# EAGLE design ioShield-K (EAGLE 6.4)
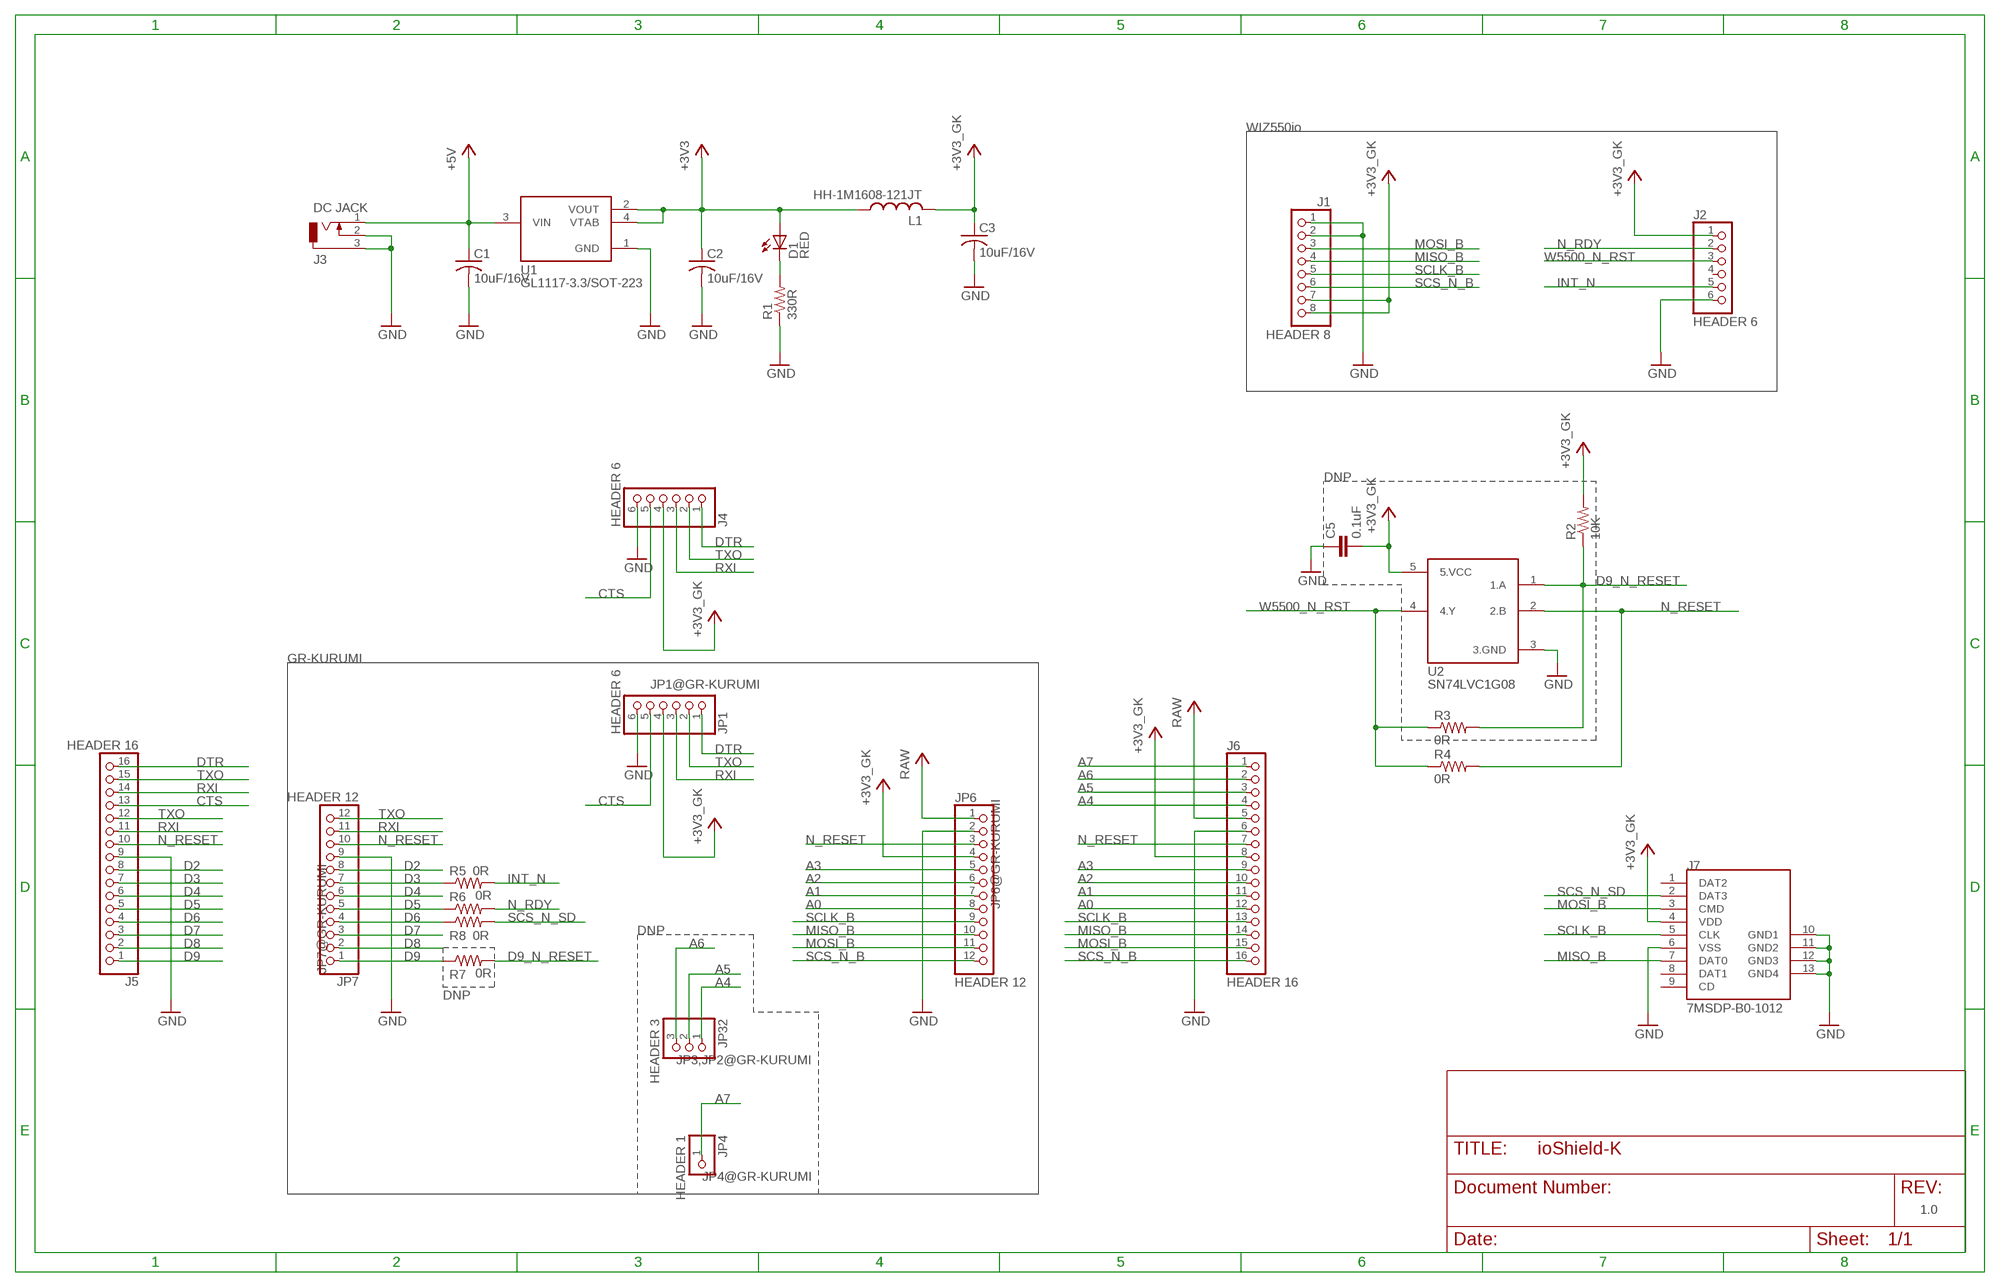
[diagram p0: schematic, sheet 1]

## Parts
C1  10uF/16V  CT-A(3216)  [CT-A(3216)]
C2  10uF/16V  CT-A(3216)  [CT-A(3216)]
C3  10uF/16V  CT-A(3216)  [CT-A(3216)]
C5  0.1uF  C1608  [C1608]
D1  RED  LED1608  [CHIP-LED1608]
J1  HEADER 8  HEADER8  [HEADER1X8]
J2  HEADER 6  HEADER6  [HEADER1X6]
J3  DC JACK  DC-005  [DC-005-PACK]
J4  HEADER 6  HEADER6  [HEADER1X6]
J5  HEADER 16  HEADER16  [HEADER1X16]
J6  HEADER 16  HEADER16  [HEADER1X16]
J7  7MSDP-B0-1012  [MICROSD_HC]
JP1  HEADER 6  HEADER6  [HEADER1X6]
JP4  HEADER 1  HEADER1  [HEADER1X1]
JP6  HEADER 12  HEADER12  [HEADER1X12]
JP7  HEADER 12  HEADER12  [HEADER1X12]
JP32  HEADER 3  HEADER3  [HEADER1X3]
L1  HH-1M1608-121JT  L1608  [L1608]
R1  330R  R1608  [R1608]
R2  10K  R1608  [R1608]
R3  0R  R1608  [R1608]
R4  0R  R1608  [R1608]
R5  0R  R1608  [R1608]
R6  0R  R1608  [R1608]
R7  0R  R1608  [R1608]
R8  0R  R1608  [R1608]
U1  GL1117-3.3/SOT-223  [SOT223_HC]
U2  SN74LVC1G08  SN74LVC08DBV  [SOT-23-5]

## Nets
+3V3: C2.+ D1.A L1.1 U1.2(VOUT) U1.4(VTAB)
+3V3_GK: C3.+ C5.2 J1.7 J1.8 J2.1 J4.4 J6.8 J7.4(VDD) JP1.4 JP6.4 L1.2 R2.2 U2.5(5.VCC)
+5V: C1.+ J3.1 U1.3(VIN)
A0: J6.12 JP6.8
A1: J6.11 JP6.7
A2: J6.10 JP6.6
A3: J6.9 JP6.5
A4: J6.4 JP32.1
A5: J6.3 JP32.2
A6: J6.2 JP32.3
A7: J6.1 JP4.1
CTS: J4.5 J5.13 JP1.5
D2: J5.8 JP7.8
D3: J5.7 JP7.7 R5.1
D4: J5.6 JP7.6
D5: J5.5 JP7.5 R6.1
D6: J5.4 JP7.4 R8.1
D7: J5.3 JP7.3
D8: J5.2 JP7.2
D9: J5.1 JP7.1 R7.1
D9_N_RESET: R2.1 R3.2 R7.2 U2.1(1.A)
DTR: J4.1 J5.16 JP1.1
GND: C1.- C2.- C3.- C5.1 J1.1 J1.2 J2.6 J3.2 J3.3 J4.6 J5.9 J6.6 J7.6(VSS) J7.10(GND1) J7.11(GND2) J7.12(GND3) J7.13(GND4) JP1.6 JP6.2 JP7.9 R1.1 U1.1(GND) U2.3(3.GND)
INT_N: J2.5 R5.2
MISO_B: J1.4 J6.14 J7.7(DAT0) JP6.10
MOSI_B: J1.3 J6.15 J7.3(CMD) JP6.11
N$3: D1.C R1.2
N_RDY: J2.2 R6.2
N_RESET: J5.10 J6.7 JP6.3 JP7.10 R4.2 U2.2(2.B)
RAW: J6.5 JP6.1
RXI: J4.3 J5.11 J5.14 JP1.3 JP7.11
SCLK_B: J1.5 J6.13 J7.5(CLK) JP6.9
SCS_N_B: J1.6 J6.16 JP6.12
SCS_N_SD: J7.2(DAT3) R8.2
TXO: J4.2 J5.12 J5.15 JP1.2 JP7.12
W5500_N_RST: J2.3 R3.1 R4.1 U2.4(4.Y)
Unconnected: J2.4 J7.1(DAT2) J7.8(DAT1) J7.9(CD)

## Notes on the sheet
- WIZ550io
- DNP
- GR-KURUMI
- JP1@GR-KURUMI
- JP6@GR-KURUMI
- DNP
- JP7@GR-KURUMI
- DNP
- JP3,JP2@GR-KURUMI
- JP4@GR-KURUMI
- 1.0

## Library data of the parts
C1-C3 = rlc_HC:CT-A(3216): CT-A(3216)
C5 = rlc_HC:C1608: C1608
D1 = rlc_HC:LED1608: LED 1608
J1 = pinheader_HC:HEADER8: HEADER 1X8 2.54mm
J2 J4 JP1 = pinheader_HC:HEADER6: HEADER 1X6 2.54mm
J3 = con-jack_HC:DC-005: DC-005
J5 J6 = pinheader_HC:HEADER16: HEADER 1X16 2.54mm
J7 = socket_HC:7MSDP-B0-1012: Micro SD Connector Part No. 7MSDP-B0-1012
JP4 = pinheader_HC:HEADER1: HEADER 1X1
JP6 JP7 = pinheader_HC:HEADER12: HEADER 1X12 2.54mm
JP32 = pinheader_HC:HEADER3: HEADER 1X3 2.54mm
L1 = rlc_HC:L1608: L1608
R1-R8 = rlc_HC:R1608: R1608
U1 = dc-dc:GL1117-3.3/SOT-223: GL1117-3.3/SOT-223
U2 = logic_HC:SN74LVC08DBV: SN74LVC1G08DBV 2Input Single AND Gate

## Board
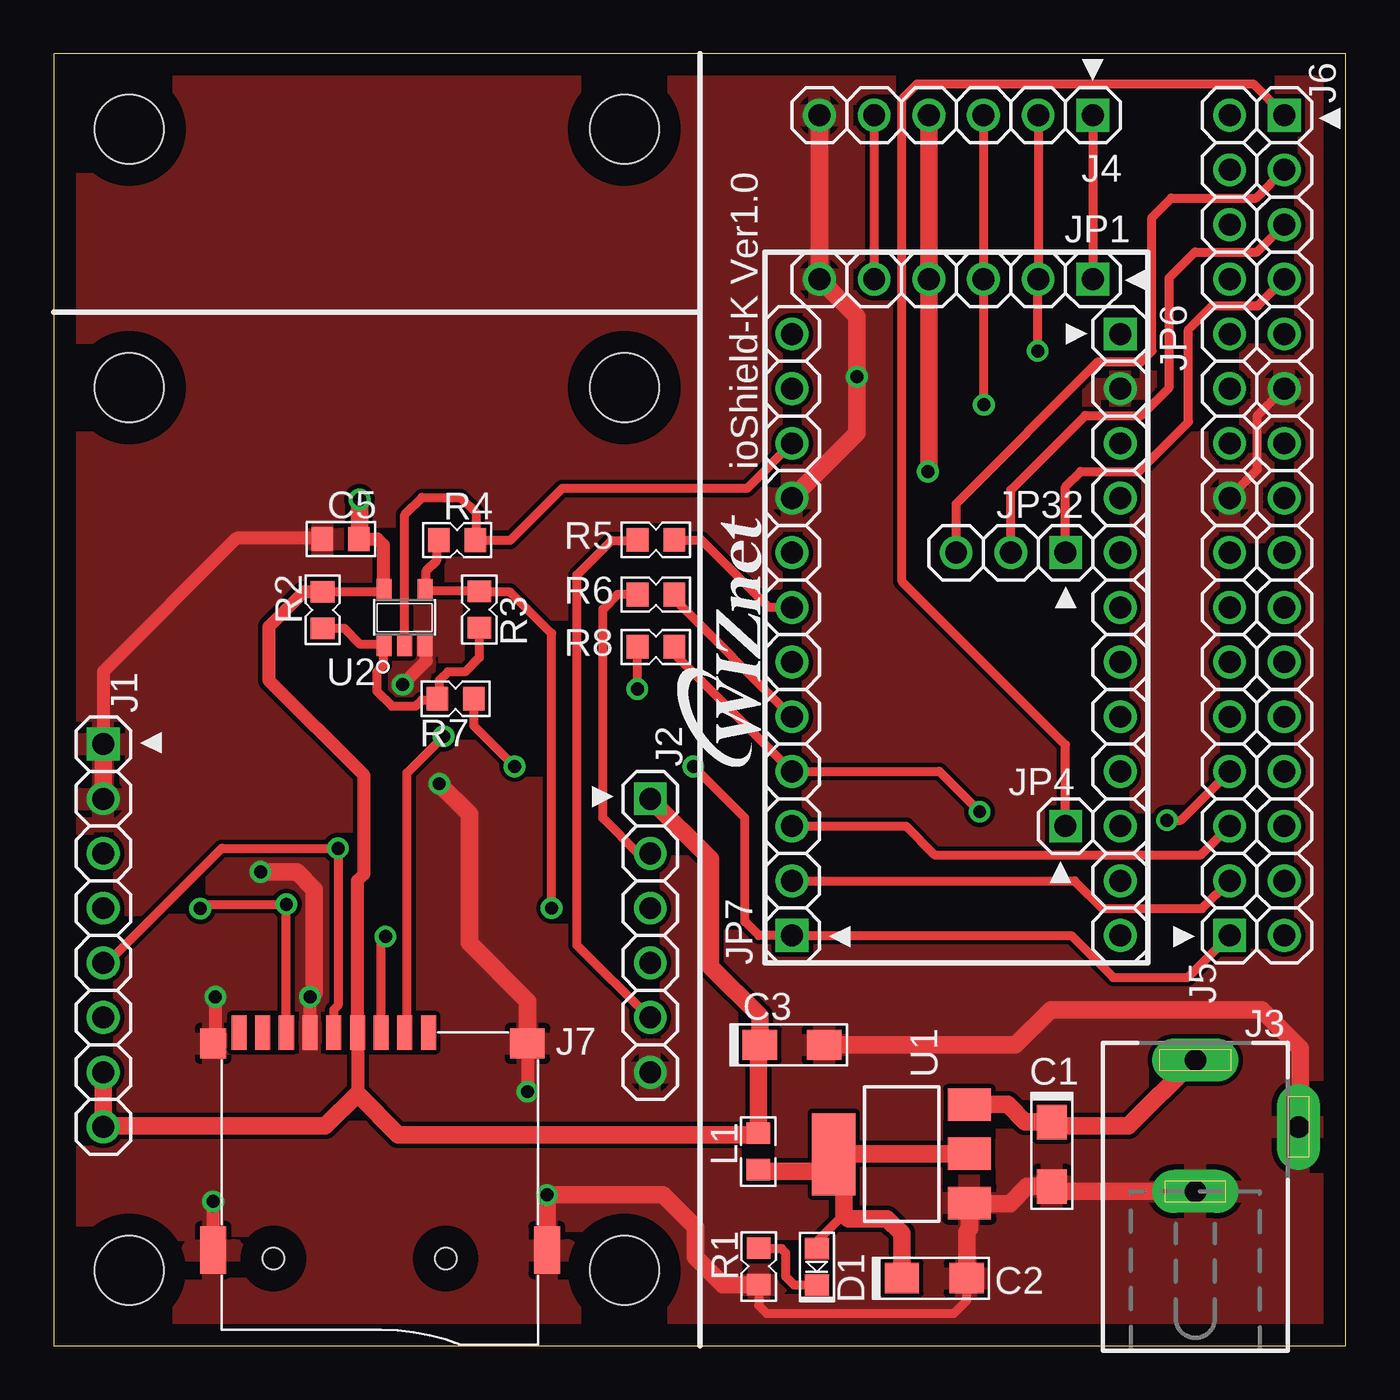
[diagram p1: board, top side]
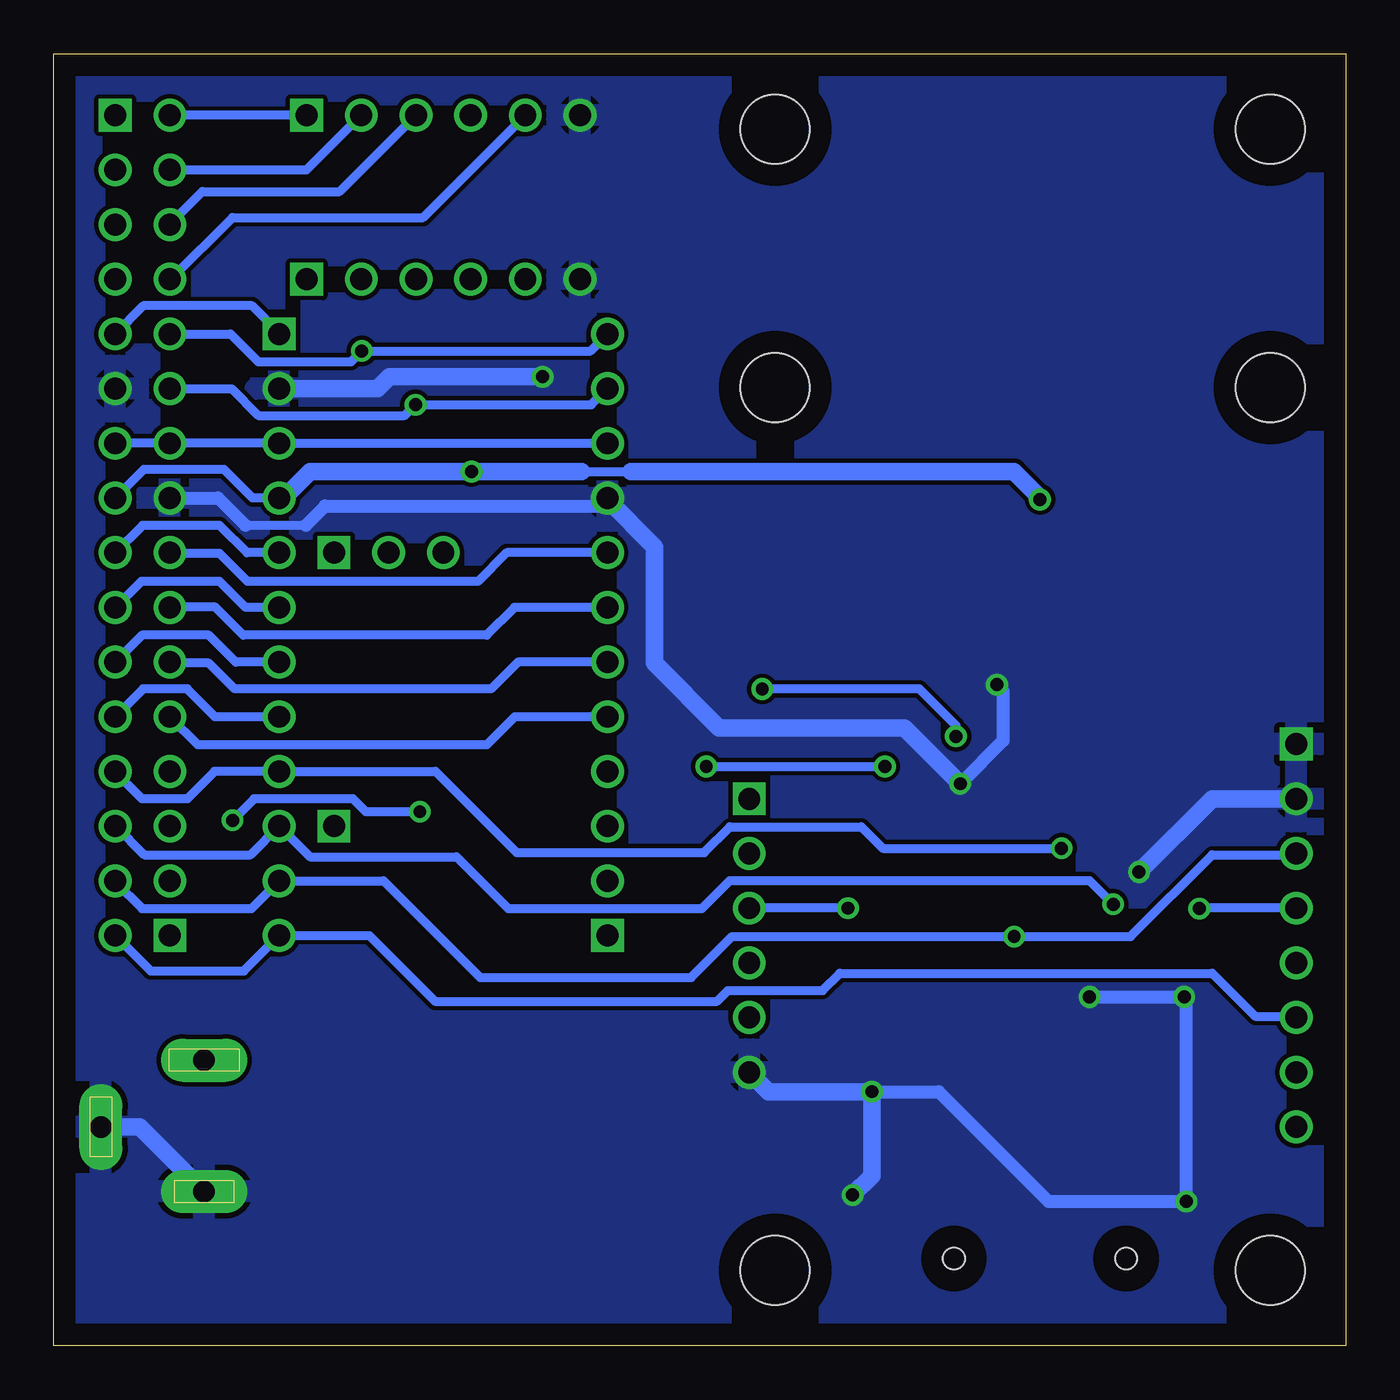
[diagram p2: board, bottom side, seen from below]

Size 60 x 60 mm. Coordinates in mm from the lower left corner, seen from the top.
Outline: 0,0 60,0 60,60 0,60 0,0
Copper layers (1*16): Top 0.035mm / dielectric 1.5mm / Bottom 0.035mm
Design rules "default *": minimum track width 10mil, minimum drill 23mil, track to track 8mil, track to pad 8mil, pad to pad 8mil, via to via 8mil, smd to smd 8mil, copper to edge 40mil, drill to drill 8mil, minimum pad ring 10mil, minimum via ring 8mil, stop-mask expansion 4mil, vias tented up to drill 0mil, thermal gap 10mil
Holes 3.2 mm at 3.5,3.5 26.5,3.5 3.5,44.5 26.5,44.5 3.5,56.5 26.5,56.5

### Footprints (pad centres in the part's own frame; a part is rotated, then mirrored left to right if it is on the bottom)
CT-A(3216) = smd 1.6 x 1.4: + -1.5,0; - 1.5,0
C1608 = smd 1 x 1.1: 1 -0.85,0; 2 0.85,0
CHIP-LED1608 = smd 1 x 1.1: A -0.85,0; C 0.85,0
HEADER1X8 = drill 1.016 square: 1 -8.89,0 | drill 1.016: 2 -6.35,0; 3 -3.81,0; 4 -1.27,0; 5 1.27,0; 6 3.81,0; 7 6.35,0; 8 8.89,0
HEADER1X6 = drill 1.016 square: 1 -6.35,0 | drill 1.016: 2 -3.81,0; 3 -1.27,0; 4 1.27,0; 5 3.81,0; 6 6.35,0
DC-005-PACK = drill 1 pad 2 long: 1 0,5.64; 2 0,-0.46; 3 4.8,2.54
HEADER1X16 = drill 1.016 square: 1 -19.05,0 | drill 1.016: 2 -16.51,0; 3 -13.97,0; 4 -11.43,0; 5 -8.89,0; 6 -6.35,0; 7 -3.81,0; 8 -1.27,0; 9 1.27,0; 10 3.81,0; 11 6.35,0; 12 8.89,0; 13 11.43,0; 14 13.97,0; 15 16.51,0; 16 19.05,0
MICROSD_HC = smd 0.7 x 1.6: 1 10.6,11.2; 2 9.5,11.2; 3 8.4,11.2; 4 7.3,11.2; 5 6.2,11.2; 6 5.1,11.2; 7 4,11.2; 8 2.9,11.2; 9 1.8,11.2 | smd 1.2 x 1.4: 10 0.6,10.7 | smd 1.6 x 1.4: 11 15.2,10.7 | smd 1.2 x 2.2: 12 16.1,1.1; 13 0.6,1.1 | hole 1: 3.4,0.7; 11.4,0.7
HEADER1X1 = drill 1.016 square: 1 0,0
HEADER1X12 = drill 1.016 square: 1 -13.97,0 | drill 1.016: 2 -11.43,0; 3 -8.89,0; 4 -6.35,0; 5 -3.81,0; 6 -1.27,0; 7 1.27,0; 8 3.81,0; 9 6.35,0; 10 8.89,0; 11 11.43,0; 12 13.97,0
HEADER1X3 = drill 1.016 square: 1 -2.54,0 | drill 1.016: 2 0,0; 3 2.54,0
L1608 = smd 1 x 1.1: 1 -0.85,0; 2 0.85,0
R1608 = smd 1 x 1.1: 1 -0.85,0; 2 0.85,0
SOT223_HC = smd 1.499 x 2.007: 1 -2.261,-3.15; 2 0.025,-3.15; 3 2.311,-3.15 | smd 3.81 x 2.007: 4 0,3.15
SOT-23-5 = smd 0.69 x 0.99: 1 -0.95,-1.29; 2 0,-1.29; 3 0.95,-1.29; 4 0.95,1.3; 5 -0.95,1.3

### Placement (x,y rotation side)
C1  46.35,8.89 270 top
C2  40.89,3.14 0 top
C3  34.29,13.97 0 top
C5  13.32,37.47 0 top
D1  35.44,3.66 270 top
J1  2.3,19.05 270 top
J2  27.7,19.05 270 top
J3  53.02,7.62 0 top
J4  41.91,57.15 180 top
J5  54.61,38.1 90 top
J6  57.15,38.1 270 top
J7  6.8,3.34 0 top
JP1  41.91,49.53 180 top
JP4  46.99,24.13 0 top
JP6  49.53,33.02 270 top
JP7  34.29,33.02 90 top
JP32  44.45,36.83 180 top
L1  32.72,9.02 90 top
R1  32.74,3.68 90 top
R2  12.48,34.17 90 top
R3  19.76,34.19 270 top
R4  18.73,37.41 0 top
R5  27.96,37.42 180 top
R6  27.96,34.88 180 top
R7  18.66,30.05 180 top
R8  27.96,32.45 180 top
U1  39.37,8.89 90 top
U2  16.3,33.82 0 top

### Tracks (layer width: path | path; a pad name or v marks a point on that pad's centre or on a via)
+3V3
  Top 0.406: D1.A 35.44,4.84 36.7,6.1
  Top 0.813: U1.2 36.25,8.91 U1.4 | L1.1 32.79,8.1 35.43,8.1 U1.4 | C2.+ 39.39,5.21 38.7,5.9 36.9,5.9 36.7,6.1 36.7,8.41 U1.4
+3V3_GK  (via drill 0.6)
  Top 0.406: R2.2 15.25,35.02 U2.5 | 14.2,37.49 C5.2
  Top 0.61: 14.1,11.7 J7.4 14.1,21.6 14.4,21.9 14.4,26.5 10,30.9 10,33.4 11.62,35.02 R2.2 | C5.2 15.04,37.47 15.3,37.2 15.3,35.16 U2.5
  Top 0.813: J1.7 J1.8 2.34,10.2 12.6,10.2 14.1,11.7 16,9.8 32.65,9.8 L1.2 32.72,13.9 C3.+ 32.79,15.31 30.5,17.6 30.5,22.6 J2.1 | J4.4 JP1.4 40.64,40.64 v40.6,40.6 | 14.2,37.49 v14.2,39.3
  Bottom 0.406: JP6.4 50.77,39.37 52.1,40.7 55.82,40.7 J6.8 | 35.5,40.6 33.2,40.6
  Bottom 0.813: JP6.4 49.33,39.37 48.1,40.6 v40.6,40.6 35.5,40.6 | v14.2,39.3 14.2,39.4 15.4,40.6 33.2,40.6
+5V
  Top 0.813: J3.1 52.96,13.26 49.9,10.2 46.55,10.2 C1.+ 45.11,10.39 44.3,11.2 U1.3
A0
  Bottom 0.406: JP6.8 52.51,29.21 53.8,30.5 55.86,30.5 J6.12
A1
  Bottom 0.406: JP6.7 51.55,31.75 52.8,33 55.9,33 J6.11
A2
  Bottom 0.406: JP6.6 51.09,34.29 52.3,35.5 55.94,35.5 J6.10
A3
  Bottom 0.406: JP6.5 51.03,36.83 52.3,38.1 55.88,38.1 J6.9
A4
  Top 0.406: JP32.1 46.99,39.89 47.7,40.6 50.4,40.6 52.7,42.9 52.7,47.2 53.8,48.3 55.92,48.3 J6.4
A5
  Top 0.406: JP32.2 44.45,39.75 47.9,43.2 50.5,43.2 51.8,44.5 51.8,49.6 53,50.8 55.88,50.8 J6.3
A6
  Top 0.406: JP32.3 41.91,39.11 48.5,45.7 50.5,45.7 51,46.2 51,52.4 51.9,53.3 55.84,53.3 J6.2
A7
  Top 0.406: JP4.1 46.99,27.91 39.4,35.5 39.4,57.9 40.1,58.6 55.7,58.6 J6.1
CTS
  Top 0.406: J4.5 JP1.5
  Bottom 0.406: J5.13 54.57,49.53 51.7,52.4 42.85,52.4 J4.5
D2
  Bottom 0.406: JP7.8 38.97,36.83 40.3,35.5 51,35.5 52.3,36.8 54.58,36.8 J5.8
D3
  Top 0.406: R5.1 30.07,37.42 33.2,34.3 JP7.7
  Bottom 0.406: JP7.7 38.61,34.29 39.9,33 51.2,33 52.5,34.3 J5.7
D4
  Bottom 0.406: JP7.6 38.45,31.75 39.7,30.5 51.6,30.5 52.8,31.7 54.56,31.7 J5.6
D5
  Top 0.406: R6.1 28.81,34.69 JP7.5
  Bottom 0.406: JP7.5 38.59,29.21 39.9,27.9 53.3,27.9 J5.5
D6  (via drill 0.6)
  Top 0.406: R8.1 28.81,32.15 JP7.4 41.13,26.67 v43,24.8 | v51.7,24.4 52.34,24.4 J5.4
  Bottom 0.406: v43,24.8 45.5,24.8 46.1,25.4 50.7,25.4 v51.7,24.4
D7
  Top 0.406: JP7.3 39.57,24.13 40.9,22.8 53.28,22.8 J5.3
D8
  Top 0.406: JP7.2 47.41,21.59 48.7,20.3 53.32,20.3 J5.2
D9  (via drill 0.6)
  Top 0.406: J5.1 52.66,17.1 49.2,17.1 47.25,19.05 JP7.1 32.75,19.05 32.1,19.7 32.1,24.5 v29.7,26.9 | v21.4,26.9 19.51,28.79 R7.1
  Bottom 0.406: v29.7,26.9 v21.4,26.9
D9_N_RESET
  Top 0.406: R2.1 13.47,33.33 14.2,32.6 15.28,32.6 U2.1 15.3,32.48 15.3,31.6 15,31.3 15,30.4 15.7,29.7 16.8,29.7 17.1,30 17.76,30 R7.2 17.9,30.14 17.9,30.9 18.3,31.3 19.1,31.3 19.76,31.96 R3.2
DTR
  Top 0.406: J4.1 JP1.1
  Bottom 0.406: J4.1 J5.16
GND  (via drill 0.6)
  Top 0.406: R1.1 32.74,1.86 33.1,1.5 41.8,1.5 42.4,2.1 C2.- | J5.9 54.61,39.41 55.9,40.7 55.9,43.2 J6.6
  Top 0.61: J7.6 v11.9,16.2 | v7.5,16.2 7.5,14.14 J7.10 | J7.13 v7.4,6.7 | J7.11 v22,11.8 | C5.1 12.44,37.5 8.5,37.5 2.3,31.3 J1.1 | U2.3 17.27,32.5 | v16.2,30.7 17.3,31.8 17.3,32.48 U2.3 | 17.2,32.48 U2.3
  Top 0.813: J3.2 46.59,7.16 C1.- 45.19,7.39 44.4,6.6 42.55,6.6 U1.1 42.52,5.42 42.4,5.3 C2.- | C3.- 44.67,13.97 46.3,15.6 56.1,15.6 57.9,13.8 57.9,10.24 J3.3 | R1.1 31.07,2.83 29.8,4.1 29.8,5.5 28.3,7 v22.9,7 J7.12 23,4.54 | J7.11 22,16 19.3,18.7 19.3,24.7 v17.9,26.1 | J4.6 JP1.6 37.3,47.8 v37.3,45 37.3,42.38 JP7.9 | J1.1 J1.2 | v9.6,22 11.3,22 12.1,21.2 12.1,16.4 v11.9,16.2
  Bottom 0.406: 48.3,38.1 51.1,38.1
  Bottom 0.61: v11.9,16.2 v7.5,16.2 7.4,16.1 v7.4,6.7 13.8,6.7 18.9,11.8 v22,11.8 | J5.9 52.37,39.37 51.1,38.1 | 48.3,38.1 47.4,39 34.66,39 JP7.9 | v16.2,30.7 15.9,30.4 15.9,28.1 v17.9,26.1
  Bottom 0.813: J3.3 56.02,10.16 J3.2 | v22.9,7 22,7.9 v22,11.8 26.8,11.8 J2.6 | J1.2 6.2,25.4 v9.6,22 | JP7.9 34.29,39.29 32.1,37.1 32.1,31.7 29.1,28.7 20.5,28.7 v17.9,26.1 | JP6.2 44.95,44.45 44.4,45 v37.3,45
  pour Bottom: -0.5,-0.5 60.5,-0.5 60.5,60.5 -0.5,60.5
  pour Top: -0.5,-0.5 60.5,-0.5 60.5,60.5 -0.5,60.5
INT_N
  Top 0.406: J2.5 27.66,15.24 24.3,18.6 24.3,35.8 25.9,37.4 27.09,37.4 R5.2
MISO_B  (via drill 0.6)
  Top 0.406: J7.7 v10.8,20.5 7,20.5 v6.8,20.3
  Bottom 0.406: v10.8,20.5 11.9,21.6 28.6,21.6 29.9,20.3 38.9,20.3 41.3,22.7 48.1,22.7 JP6.10 50.86,22.8 55.8,22.8 57.13,24.13 J6.14 | J1.4 6.78,20.32 v6.8,20.3
MOSI_B  (via drill 0.6)
  Top 0.406: J7.3 15.2,18.8 v15.4,19
  Bottom 0.406: J1.3 2.36,22.8 6.2,22.8 10,19 v15.4,19 28.5,19 30.4,17.1 40.2,17.1 44.69,21.59 JP6.11 50.82,20.3 55.9,20.3 57.15,21.55 J6.15
N$3
  Top 0.406: D1.C 34.39,2.81 34,3.2 34,4.3 33.8,4.5 32.77,4.5 R1.2
N_RDY
  Top 0.406: J2.2 27.14,22.86 25.5,24.5 25.5,34.2 26.2,34.9 27.09,34.9 R6.2
N_RESET
  Top 0.406: JP7.10 32.2,39.81 23.61,39.81 21.2,37.4 19.59,37.4 R4.2 19.6,37.44 19.6,38.7 18.9,39.4 17.1,39.4 16.3,38.59 U2.2
  Bottom 0.406: JP7.10 JP6.3 J5.10 J6.7
RAW
  Bottom 0.406: JP6.1 49.53,47.03 50.8,48.3 55.84,48.3 J6.5
RXI  (via drill 0.6)
  Top 0.406: J4.3 JP1.3 43.2,49.51 v43.2,43.7
  Bottom 0.406: J5.14 54.61,52.09 53.1,53.6 46.73,53.6 J4.3 | J5.11 51.75,44.45 50.5,43.2 43.7,43.2 v43.2,43.7 35.04,43.7 JP7.11
SCLK_B  (via drill 0.6)
  Top 0.406: J1.5 2.62,18.1 2.8,18.1 7.8,23.1 v13.2,23.1 13.2,15.8 13,15.6 J7.5
  Bottom 0.406: v13.2,23.1 21.5,23.1 22.5,24.1 28.6,24.1 29.8,22.9 38.5,22.9 42.27,26.67 JP6.9 52.53,26.67 53.8,25.4 55.9,25.4 57.15,26.65 J6.13
SCS_N_B
  Bottom 0.406: J1.6 2.36,15.3 4.2,15.3 6.2,17.3 23.5,17.3 24.3,16.5 28.7,16.5 29.2,16 42.3,16 45.35,19.05 JP6.12 51.18,17.4 55.5,17.4 J6.16
SCS_N_SD  (via drill 0.6)
  Top 0.406: v27.1,30.5 R8.2 | J7.2 16.4,14.64 16.4,26.6 v18.1,28.3
  Bottom 0.406: v27.1,30.5 19.8,30.5 18.1,28.8 v18.1,28.3
TXO  (via drill 0.6)
  Top 0.406: J4.2 JP1.2 45.7,49.51 v45.7,46.2
  Bottom 0.406: J5.15 48.26,54.61 J4.2 | J5.12 51.79,46.99 50.5,45.7 46.2,45.7 v45.7,46.2 35.08,46.2 JP7.12
W5500_N_RST  (via drill 0.6)
  Top 0.406: v23.12,20.32 23.12,33.08 21.2,35 19.8,35 R3.1 17.32,35.04 U2.4 17.3,35.17 17.3,36 17.8,36.5 17.8,37.34 R4.1
  Bottom 0.406: v23.12,20.32 J2.3

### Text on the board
tPlace: ioShield-K Ver1.0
